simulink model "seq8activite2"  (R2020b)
settings: Solver=VariableStepAuto  StartTime=0.0  StopTime=inf  RelTol=1e-3  EnableMultiTasking=on

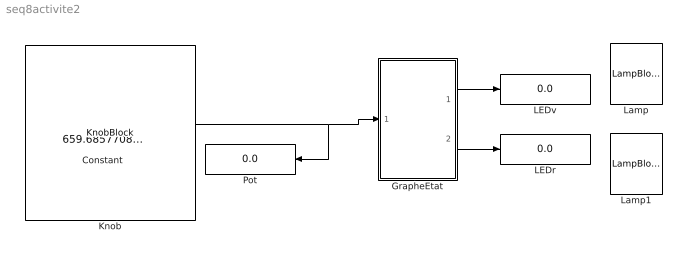
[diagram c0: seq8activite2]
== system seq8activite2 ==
  Constant : Constant  Value=659.6857708740236
  GrapheEtat : Stateflow chart  TreatAsAtomicUnit=on
  Knob : KnobBlock  ScaleMax=1023
  LEDr : Display
  LEDv : Display
  Lamp : LampBlock
  Lamp1 : LampBlock
  Pot : Display
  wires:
  Constant/1 -> GrapheEtat/1(pot), Pot/1
  GrapheEtat/1(LEDv) -> LEDv/1
  GrapheEtat/2(LEDr) -> LEDr/1

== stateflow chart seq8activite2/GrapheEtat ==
  data: pot input; LEDv output; LEDr output
